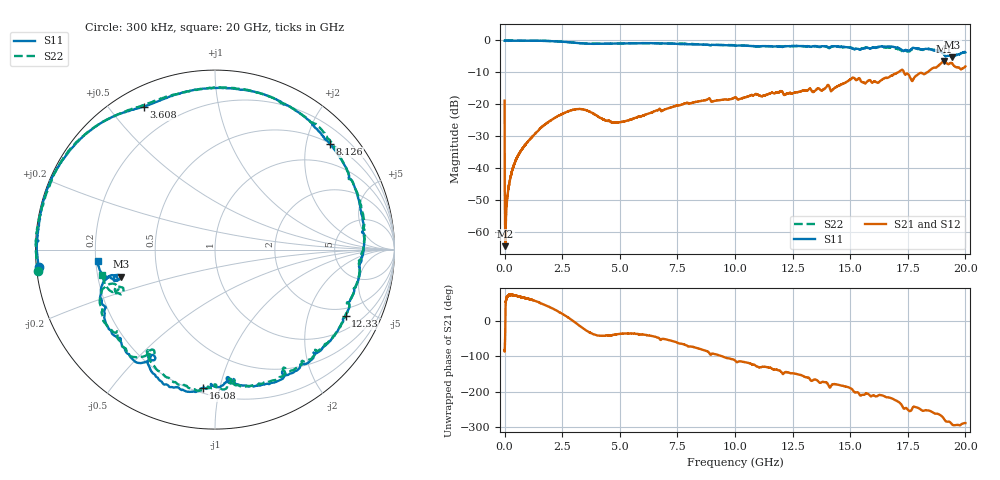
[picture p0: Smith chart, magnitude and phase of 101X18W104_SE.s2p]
!{101X18W104_SE}
!Johanson Technology Inc.
!www.johansontechnology.com
!Test Board Conditions:
!Substrate Type  RO4350B
!Substrate Thickness  21 mil
!Substrate Dk  3.66
!TL Type: GCPW
!TL Trace Width  40 mil
!TL Gap  20 mil
!PART MODE SINGLE ENDED (AKA BYPASS)
!DUT TOPOLOGY	SERIES-SHUNT
!Mounting Pad LxW  120x40 mil
! Created Wed Oct 27 11:10:21 2021
# hz S ma R 50
! 2 Port Network Data from SP1.SP block
! freq  magS11  angS11  magS21  angS21  magS12  angS12  magS22  angS22
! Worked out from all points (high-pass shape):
!   20001 points, 300 kHz to 20 GHz, reference 50 ohm
!   highest |S21| = -6.39 dB at 19.07 GHz (marker M1); lowest = -64.3 dB at 30.3 MHz (marker M2)
!   |S21| within 3 dB of the highest: 17.2 GHz to 17.3 GHz (100.6 MHz wide, 0.583 % of centre); 18.44 GHz to end of sweep
!   lowest |S11| = -5.3 dB at 19.44 GHz (marker M3), VSWR 3.40, Z = 15 - j6.42 ohm
!   |S11| at or under -10 dB: nowhere
!   |S22| runs from -5.1 to 0.0 dB; largest |S21 - S12| = 0.013
!   S11 on the Smith chart (normalised r, x): 300 kHz: 0.01, -0.05; 3.608 GHz: 0.08, +0.62; 8.126 GHz: 0.51, +2.48; 12.33 GHz: 1.57, -3.50; 16.08 GHz: 0.23, -0.89; 20 GHz: 0.21, -0.04
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300000  0.988 -174.3  0.1148 -82.7  0.1152 -83.5  0.9931 -173.0
3.03e7  0.9941 179.4  0.0006078 -7.3  0.0006125 -11.1  0.9999 179.5
1.073e8  0.9924 178.1  0.003173 65.1  0.003153 67.4  0.9995 178.0
2.063e8  0.9924 176.3  0.00585 73.2  0.005896 71.7  0.9977 176.3
3.623e8  0.9905 173.4  0.01026 72.4  0.01014 71.9  0.9976 173.6
8.813e8  0.9944 164.5  0.02302 64.2  0.02311 64.3  0.9905 164.3
2.0653e9  0.9732 142.3  0.05799 35.2  0.05795 35.1  0.9758 142.3
3.3343e9  0.901 120.1  0.08428 -17.8  0.08463 -17.9  0.9042 118.9
3.6083e9  0.8882 116.4  0.0793 -29.7  0.07957 -29.8  0.8971 115.0
4.8103e9  0.8957 99.1  0.05221 -38.5  0.05236 -38.6  0.8942 99.7
6.6673e9  0.9017 66.0  0.08213 -47.5  0.08226 -47.8  0.9031 67.0
8.1263e9  0.8701 42.6  0.1056 -72.8  0.1049 -72.6  0.8809 42.6
1.00003e10  0.8307 7.3  0.1293 -111.6  0.1301 -111.5  0.8377 8.8
1.23343e10  0.8166 -27.0  0.1494 -145.6  0.1474 -145.3  0.8164 -26.6
1.33343e10  0.8017 -46.3  0.1624 -169.3  0.1631 -168.9  0.7949 -45.0
1.51053e10  0.7513 -81.5  0.2623 165.4  0.2612 164.9  0.755 -82.1
1.60823e10  0.773 -94.9  0.2296 147.6  0.2299 147.9  0.7682 -92.8
1.66673e10  0.8023 -107.0  0.2657 144.1  0.2642 146.3  0.7747 -106.0
1.84253e10  0.7354 -145.3  0.3349 107.0  0.3373 106.8  0.7379 -147.5
1.90733e10  0.5977 -166.2  0.4791 83.7  0.4772 83.9  0.6106 -161.9
1.94403e10  0.5456 -164.0  0.4316 67.2  0.4281 67.1  0.5549 -157.1
2e10  0.6527 -174.9  0.395 72.0  0.3944 71.1  0.6471 -168.0
